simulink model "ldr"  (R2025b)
settings: Solver=FixedStepAuto  StartTime=0.0  StopTime=inf  RelTol=1e-3  EnableMultiTasking=on
libraries: arduinolib x2

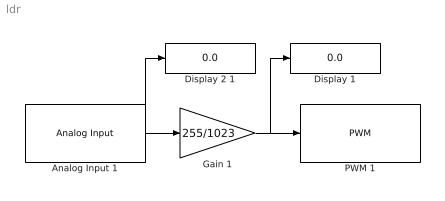
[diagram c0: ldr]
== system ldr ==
  Analog Input 1 : arduinolib/Analog Input  pinNumber=0  ReadResultsOnly=off  ConversionTriggerSource=Software  ExternalTriggerType=uint32( 0 )  OutputDataType=uint16  EnableConversionCompleteNotify=off  EnableOuputStatus=off  SampleTime=0.01  blockPlatform=arduino
  Display 1 : Display
  Display 2 1 : Display
  Gain 1 : Gain  Gain=255/1023
  PWM 1 : arduinolib/PWM  pinNumber=9  frequencyType=Default  desiredFrequency=490.2  achievableFrequency=490.2
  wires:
  Analog Input 1/1 -> Display 2 1/1, Gain 1/1
  Gain 1/1 -> Display 1/1, PWM 1/1
